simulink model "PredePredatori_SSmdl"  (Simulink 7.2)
settings: Solver=ode45  StartTime=0.0  StopTime=10.0  RelTol=1e-3
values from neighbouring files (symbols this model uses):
  D = zeros(2,2)    [Exercises04a.m]
  x0sl = x0-xe    [Exercises04a.m]
undefined symbols (not defined in the file or in its folder): A, B, C

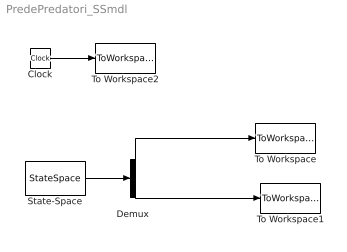
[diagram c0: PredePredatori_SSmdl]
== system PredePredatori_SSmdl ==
  Clock : Clock
  Demux : Demux  Outputs=2
  State-Space : StateSpace  A=A  B=B  C=C  D=D  X0=x0sl
  To Workspace : ToWorkspace  VariableName=x1ss  SampleTime=-1  SaveFormat=Array
  To Workspace1 : ToWorkspace  VariableName=x2ss  SampleTime=-1  SaveFormat=Array
  To Workspace2 : ToWorkspace  VariableName=time  SampleTime=-1  SaveFormat=Array
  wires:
  Demux/1 -> To Workspace/1
  Demux/2 -> To Workspace1/1
  Clock/1 -> To Workspace2/1
  State-Space/1 -> Demux/1
